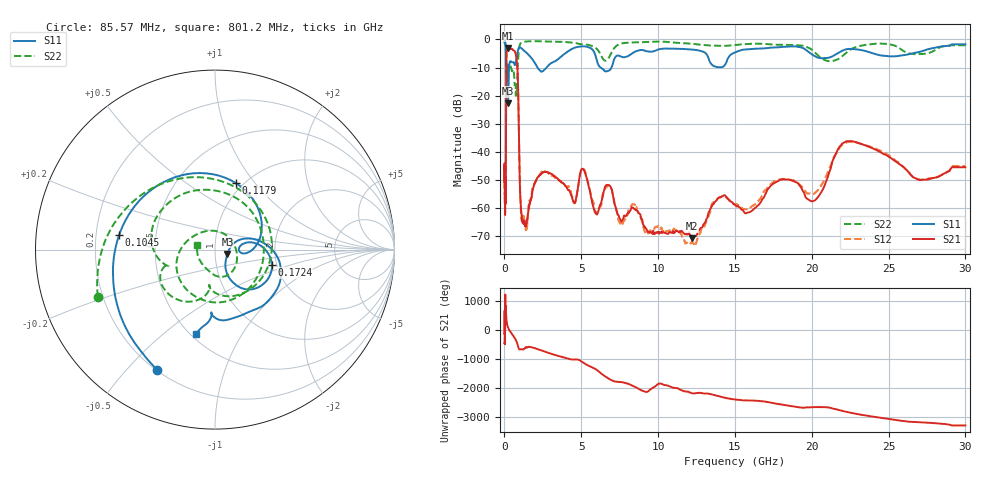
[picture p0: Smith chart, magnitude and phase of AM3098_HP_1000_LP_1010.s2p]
! Date/Time: Thu, Feb 28, 2019 8:40 AM
! Network Analyzer: Agilent Technologies E8364B Rev: A.07.50.67
! Sweep from 0.010 to 30.000 GHz, 1601 Points, Sweep Type: LOG
! Power Supply: 5.023 V, 0.002 A
# Hz S DB R 50
!freq MagS11 AngS11 MagS21 AngS21 MagS12 AngS12 MagS22 AngS22
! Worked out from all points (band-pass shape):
!   1601 points, 10 MHz to 30 GHz, reference 50 ohm
!   highest |S21| = -3.05 dB at 241.1 MHz (marker M1); lowest = -70.7 dB at 12.19 GHz (marker M2)
!   |S21| within 3 dB of the highest: 128 MHz to 770.7 MHz (642.7 MHz wide, 143 % of centre)
!   lowest |S11| = -22.7 dB at 238.7 MHz (marker M3), VSWR 1.16, Z = 57.4 - j2.83 ohm
!   |S11| at or under -10 dB: 191.4 MHz to 301.7 MHz (110.3 MHz wide, 44.7 % of centre); 2.154 GHz to 2.737 GHz (582.4 MHz wide, 23.8 % of centre); 6.267 GHz to 6.964 GHz (696.4 MHz wide, 10.5 % of centre)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
!   |S22| runs from -20.0 to -0.6 dB; largest |S21 - S12| = 0.012
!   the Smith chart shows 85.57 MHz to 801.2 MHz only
!   S11 on the Smith chart (normalised r, x): 85.57 MHz: 0.20, -0.61; 104.5 MHz: 0.30, +0.07; 117.9 MHz: 0.93, +0.81; 172.4 MHz: 1.88, -0.36; 801.2 MHz: 0.53, -0.65
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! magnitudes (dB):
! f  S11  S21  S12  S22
! 10 MHz  -0.3  -44.9  -44.6  -0.6
! 38.04 MHz  -0.5  -60.7  -61.8  -0.9
! 85.57 MHz  -2.6  -56.9  -49.8  -3.0
! 104.5 MHz  -5.4  -27.8  -28.1  -6.8
! 117.9 MHz  -8.2  -11.2  -11.2  -10.1
! 144.7 MHz  -16.8  -4.2  -4.2  -13.1
! 172.4 MHz  -9.7  -3.7  -3.7  -9.1
! 238.7 MHz  -22.7  -3.1  -3.0  -11.3
! 241.1 MHz  -22.6  -3.1  -3.0  -11.2
! 550.5 MHz  -8.0  -3.7  -3.7  -10.6
! 801.2 MHz  -6.4  -7.3  -7.3  -19.9
! 1.104 GHz  -3.1  -61.7  -63.5  -1.2
! 1.424 GHz  -4.6  -65.4  -67.8  -0.7
! 2.084 GHz  -9.3  -49.8  -49.8  -0.6
! 4.525 GHz  -3.0  -58.0  -58.3  -1.1
! 5.128 GHz  -2.4  -46.2  -45.9  -1.7
! 7.926 GHz  -6.1  -62.5  -63.5  -1.2
! 12.19 GHz  -3.6  -70.7  -72.0  -1.5
! 14.02 GHz  -9.9  -56.0  -56.2  -2.3
! 20.2 GHz  -6.0  -57.2  -54.6  -4.6
! 22.56 GHz  -3.3  -36.1  -36.4  -3.5
! 30 GHz  -1.7  -45.4  -45.0  -2.1
